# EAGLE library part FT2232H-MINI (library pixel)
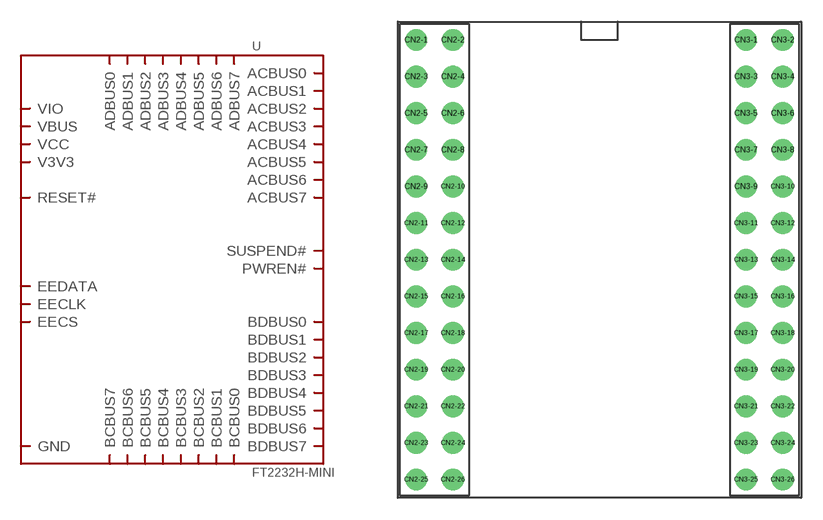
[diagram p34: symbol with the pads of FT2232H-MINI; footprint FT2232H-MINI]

Designator prefix -

## FT2232H-MINI  [FT2232H-MINI]
CN2-1  V3V3
CN2-2  GND
CN2-3  V3V3
CN2-4  GND
CN2-5  V3V3
CN2-6  GND
CN2-7  ADBUS0
CN2-8  RESET#
CN2-9  ADBUS2
CN2-10  ADBUS1
CN2-11  VIO
CN2-12  ADBUS3
CN2-13  ADBUS5
CN2-14  ADBUS4
CN2-15  ADBUS7
CN2-16  ADBUS6
CN2-17  ACBUS1
CN2-18  ACBUS0
CN2-19  ACBUS3
CN2-20  ACBUS2
CN2-21  VIO
CN2-22  ACBUS4
CN2-23  ACBUS6
CN2-24  ACBUS5
CN2-25  SUSPEND#
CN2-26  ACBUS7
CN3-1  VBUS
CN3-2  GND
CN3-3  VCC
CN3-4  GND
CN3-5  EECS
CN3-6  EECLK
CN3-7  EEDATA
CN3-8  PWREN#
CN3-9  BCBUS7
CN3-10  BCBUS6
CN3-11  BCBUS5
CN3-12  VIO
CN3-13  BCBUS4
CN3-14  BCBUS3
CN3-15  BCBUS2
CN3-16  BCBUS1
CN3-17  BCBUS0
CN3-18  BDBUS7
CN3-19  BDBUS6
CN3-20  BDBUS5
CN3-21  BDBUS4
CN3-22  VIO
CN3-23  BDBUS3
CN3-24  BDBUS2
CN3-25  BDBUS1
CN3-26  BDBUS0

## Footprint FT2232H-MINI (pad centres in mm)
drill 1: CN2-1 -12.7,15.24; CN2-2 -10.16,15.24; CN2-3 -12.7,12.7; CN2-4 -10.16,12.7; CN2-5 -12.7,10.16; CN2-6 -10.16,10.16; CN2-7 -12.7,7.62; CN2-8 -10.16,7.62; CN2-9 -12.7,5.08; CN2-10 -10.16,5.08; CN2-11 -12.7,2.54; CN2-12 -10.16,2.54; CN2-13 -12.7,0; CN2-14 -10.16,0; CN2-15 -12.7,-2.54; CN2-16 -10.16,-2.54; CN2-17 -12.7,-5.08; CN2-18 -10.16,-5.08; CN2-19 -12.7,-7.62; CN2-20 -10.16,-7.62; CN2-21 -12.7,-10.16; CN2-22 -10.16,-10.16; CN2-23 -12.7,-12.7; CN2-24 -10.16,-12.7; CN2-25 -12.7,-15.24; CN2-26 -10.16,-15.24; CN3-1 10.16,15.24; CN3-2 12.7,15.24; CN3-3 10.16,12.7; CN3-4 12.7,12.7; CN3-5 10.16,10.16; CN3-6 12.7,10.16; CN3-7 10.16,7.62; CN3-8 12.7,7.62; CN3-9 10.16,5.08; CN3-10 12.7,5.08; CN3-11 10.16,2.54; CN3-12 12.7,2.54; CN3-13 10.16,0; CN3-14 12.7,0; CN3-15 10.16,-2.54; CN3-16 12.7,-2.54; CN3-17 10.16,-5.08; CN3-18 12.7,-5.08; CN3-19 10.16,-7.62; CN3-20 12.7,-7.62; CN3-21 10.16,-10.16; CN3-22 12.7,-10.16; CN3-23 10.16,-12.7; CN3-24 12.7,-12.7; CN3-25 10.16,-15.24; CN3-26 12.7,-15.24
